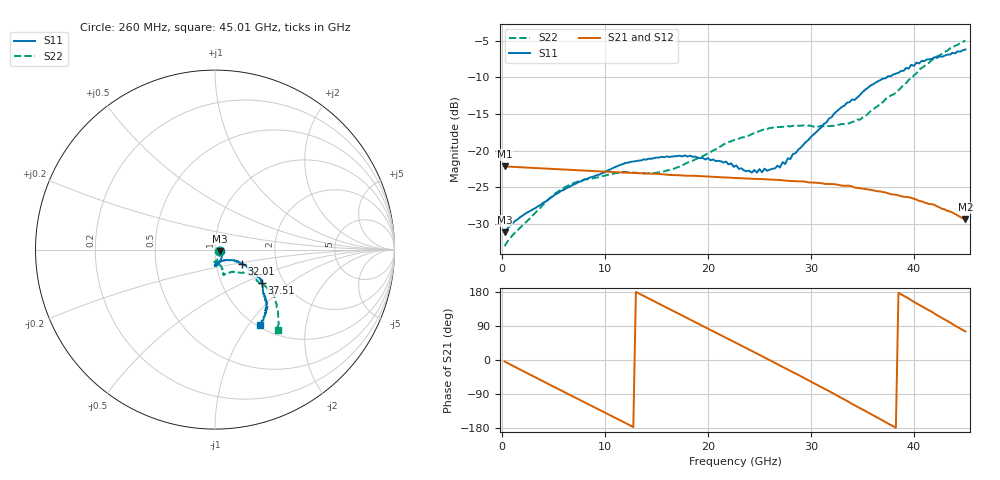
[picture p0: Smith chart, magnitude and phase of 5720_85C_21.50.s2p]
! Device:  ADRF5720
! Description: 0.5dB LSB GaAs MMIC 6-bit Digital Attenuator
! Frequency:  0.000009 -  40 GHz
! Ports:
!	RF1	= Port 1
!	RF2	= Port 2
! Vdd:  3.3 Volt
! Vss:  -3.3 Volt
! Control:  0/3.3 Volt
! State:  21.50 dB attenuation
! Data:  The device was measured using G-S-G Probes on a matrix board.
!  Data was collected using an calibrated 4 port network analyzer.
!  The reference plane for this measurement is at the launchers.
! Note:  Analog Devices supplies this data as a sample of measured data
!  for this product.  Your particular data for this product may vary.
!  Data was taken at 85 degrees C.
!  Analog Devices reserves the right to change this data at anytime.
# GHZ S DB R 45.0
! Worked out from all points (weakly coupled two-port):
!   180 points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, 260 MHz to 45.01 GHz, reference 45 ohm
!   highest |S21| = -22.17 dB at 260 MHz (marker M1); lowest = -29.4 dB at 45.01 GHz (marker M2)
!   lowest |S11| = -31.2 dB at 260 MHz (marker M3), VSWR 1.06, Z = 47.4 - j0.762 ohm
!   |S11| at or under -10 dB: start of sweep to 37.37 GHz
!   |S22| runs from -33.1 to -4.9 dB; largest |S21 - S12| = 0.00038
!   S11 on the Smith chart (normalised r, x): 260 MHz: 1.05, -0.02; 32.01 GHz: 1.33, -0.21; 37.51 GHz: 1.55, -0.65; 45.01 GHz: 1.03, -1.14
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0.26  -31.16 -16.9  -22.17 -3.9  -22.16 -3.9  -33.08 -22.2
1.26  -29.65 -3.6  -22.26 -18.2  -22.24 -18.1  -31.24 -14.4
4.76  -26.45 -38.1  -22.51 -66.8  -22.49 -66.7  -26.37 -65.9
7.76  -24.18 -55.7  -22.72 -108.1  -22.71 -108.0  -24.08 -83.2
12.01  -21.70 -74.7  -23.02 -166.5  -23.00 -166.4  -22.96 -92.4
15.26  -20.96 -85.0  -23.22 148.3  -23.21 148.5  -22.98 -86.2
18.26  -20.70 -90.3  -23.45 107.1  -23.44 107.2  -21.52 -75.7
22.76  -22.03 -83.9  -23.76 44.6  -23.75 44.8  -18.49 -69.3
24.26  -23.03 -75.8  -23.87 24.0  -23.86 24.2  -17.77 -69.9
27.01  -22.32 -50.3  -24.03 -14.7  -24.02 -14.4  -16.79 -70.5
27.26  -21.59 -46.5  -24.08 -18.3  -24.07 -18.1  -16.75 -71.2
27.51  -21.85 -45.5  -24.12 -21.7  -24.10 -21.4  -16.78 -70.6
27.76  -21.07 -41.8  -24.14 -25.2  -24.12 -24.9  -16.66 -71.4
28.01  -21.17 -42.1  -24.17 -28.7  -24.16 -28.5  -16.71 -71.0
30.26  -17.82 -30.2  -24.38 -60.6  -24.37 -60.4  -16.73 -69.7
32.01  -15.45 -27.3  -24.58 -85.7  -24.56 -85.5  -16.63 -63.9
34.76  -12.42 -30.2  -25.15 -126.6  -25.13 -126.3  -15.80 -49.2
37.51  -9.83 -35.4  -25.86 -168.0  -25.85 -167.6  -12.76 -35.3
37.76  -9.84 -35.7  -25.96 -171.6  -25.94 -171.2  -12.47 -35.4
41.51  -7.53 -47.2  -27.32 130.7  -27.30 131.0  -7.96 -37.2
43.51  -6.89 -51.4  -28.34 99.0  -28.31 99.5  -6.05 -45.1
45.01  -6.19 -59.3  -29.43 75.2  -29.43 75.5  -4.95 -52.0
